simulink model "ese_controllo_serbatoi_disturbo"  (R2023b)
settings: Solver=ode45  StartTime=0.0  StopTime=200  RelTol=1e-3  EnableMultiTasking=on
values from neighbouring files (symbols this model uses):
  k = [0:0.1:8]    [ese_controllo_serbatoi.m]

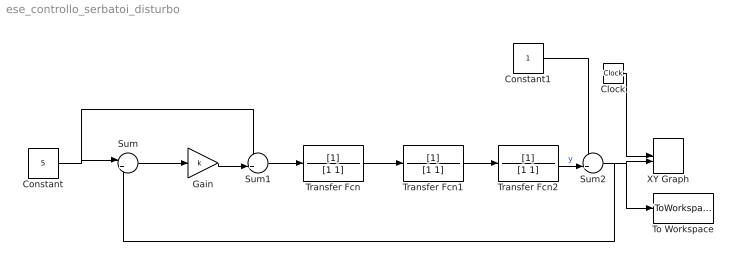
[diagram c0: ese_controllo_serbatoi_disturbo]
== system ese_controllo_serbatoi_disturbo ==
  Clock : Clock
  Constant : Constant  Value=5
  Constant1 : Constant
  Gain : Gain  Gain=k
  Sum : Sum  Inputs=|+-
  Sum1 : Sum  Inputs=++|
  Sum2 : Sum  Inputs=++|
  To Workspace : ToWorkspace  VariableName=y  SampleTime=-1
  Transfer Fcn : TransferFcn  Denominator=[1 1]
  Transfer Fcn1 : TransferFcn  Denominator=[1 1]
  Transfer Fcn2 : TransferFcn  Denominator=[1 1]
  XY Graph : Record  FileSettingsInternal="{\"entries\":[{\"content\":{\"excelSettings\":{\"content\":{},\"type\":\"Streamout.ExcelSettings\"}},\"type\":\"Streamout.FileSettingStorage\",\"uuid\":\"\"}],\"packageUris\":[\"http:\\/\\/schema.mathworks.com\\/mf0\\/streamout_blocks\\/R2020a\"],\"version\":\"1.0\"}"  Layout=[1 1]  SignalsInternal="{\"entries\":[{\"content\":{\"signals\":[{\"content\":{\"blockPath\":[],\"dimensions\":[1],\"domain\":\"\",\"lineColor\":\"#a2142f\",\"plots\":[ 1 ],\"port\":1,\"signalID\":1,\"signalName\":\"XY Graph:1\"},\"type\":\"RecordBlkView.Signal\",\"uuid\":\"\"},{\"content\":{\"blockPath\":[],\"dimensions\":[1],\"domain\":\"\",\"lineColor\":\"#139fff\",\"plots\":[ 1 ],\"port\":2,\"signalID\":2,\"signalName\":\"XY Graph:2\"},\"type\":\"RecordBlkView.Signal\",\"uuid\":\"\"}]}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"  VisualizationBindings="{\"xyplotplugin\":{\"info\":[{\"series\":[{\"bindingParametersList\":[{\"parameter\":\"X-Axis\",\"signalID\":1,\"signalName\":\"XY Graph:1\"},{\"parameter\":\"Y-Axis\",\"signalID\":2,\"signalName\":\"XY Graph:2\"}],\"seriesID\":0}],\"subplotID\":1}]}}"  CompatibilityTag=XY  st=0.1
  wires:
  Transfer Fcn/1 -> Transfer Fcn1/1
  Transfer Fcn1/1 -> Transfer Fcn2/1
  Clock/1 -> XY Graph/1
  Constant/1 -> Sum/1, Sum1/1
  Sum/1 -> Gain/1
  Gain/1 -> Sum1/2
  Sum1/1 -> Transfer Fcn/1
  Transfer Fcn2/1 -> Sum2/2  "y"
  Sum2/1 -> Sum/2, To Workspace/1, XY Graph/2
  Constant1/1 -> Sum2/1
